FUNCTION "ZWPH" : VOID
TITLE =
VERSION : 0.1


VAR_INPUT
  EIN : BOOL ;
  SW : REAL ;
  IW : REAL ;
  SH : REAL ;
END_VAR
VAR_IN_OUT
  STG : BOOL ;
END_VAR
VAR_TEMP
  ER : REAL ;
  SP : REAL ;
END_VAR
BEGIN
NETWORK
TITLE =

      UN    #EIN;
      R     #STG;
      BEB   ;
      L     #SW;
      L     #IW;
      -R    ;
      T     #ER;
      L     5.000000e-003;
      L     #SH;
      *R    ;
      L     #SW;
      *R    ;
      T     #SP;

      L     #SP;
      L     -1.000000e+000;
      *R    ;
      L     #ER;
      TAK   ;
      <R    ;
      R     #STG;
      BEB   ;
      L     #ER;
      L     #SP;
      >R    ;
      S     #STG;








END_FUNCTION

